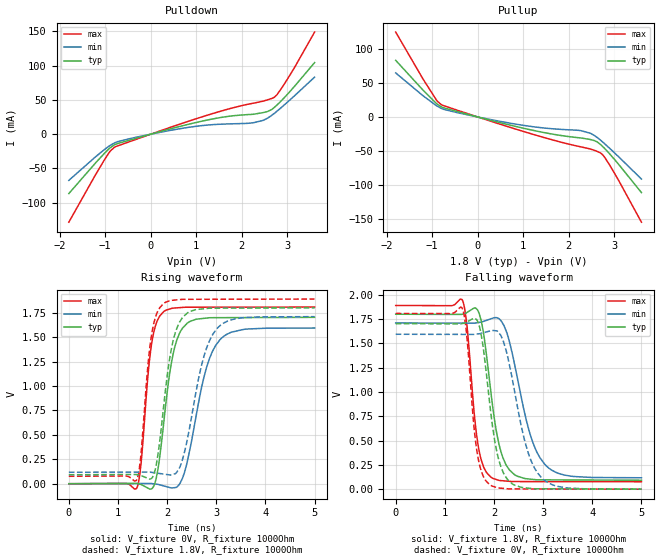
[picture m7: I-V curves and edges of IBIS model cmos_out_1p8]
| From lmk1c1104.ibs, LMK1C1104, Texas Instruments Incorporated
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[Model]   cmos_out_1p8
Model_type   Output
Polarity   Non-Inverting
Vmeas = 0.9
Vref = 0
Cref = 5pF
Rref = 100000
|   typ   min   max
C_comp   2.527pF   2.231pF   2.947pF
[Voltage Range]   1.8   1.71   1.89
[Temperature Range]   25   150   -40
[Pullup Reference]   1.8   1.71   1.89
[Pulldown Reference]   0   -0   0
[Power Clamp Reference]   1.8   1.71   1.89
[GND Clamp Reference]   0   0   0
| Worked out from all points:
|   slope of the pulldown table from 0 to 0.27 V, typ, clamps not added: 55 ohm
|   slope of the pullup table from 0 to 0.27 V, typ, clamps not added: 58.1 ohm
|   falling waveform, V_fixture 1.8V, R_fixture 1000Ohm: 20-80 % time 288ps typ, 452ps min, 202ps max; typ from 1.8 V to 0.092 V
|   rising waveform, V_fixture 0V, R_fixture 1000Ohm: 20-80 % time 272ps typ, 409ps min, 193ps max; typ from 0 V to 1.7 V
|   rising waveform, V_fixture 1.8V, R_fixture 1000Ohm: 20-80 % time 270ps typ, 402ps min, 194ps max; typ from 0.092 V to 1.8 V
|   falling waveform, V_fixture 0V, R_fixture 1000Ohm: 20-80 % time 273ps typ, 419ps min, 193ps max; typ from 1.7 V to 0 V
[Pulldown]
|   Voltage   I(typ)   I(min)   I(max)
-1.8V     -86.73mA   -67.44mA   -128.5mA
-1.012V   -27.53mA   -22.15mA   -36.77mA
-887.4mV  -19.56mA   -16.21mA   -24.46mA
-790.2mV  -15.19mA   -12.58mA   -18.76mA
840.6mV   14.63mA    10.07mA    19.14mA
1.597V    24.97mA    14.72mA    34.7mA
2.266V    29.19mA    16.87mA    45.33mA
2.471V    31.52mA    20.17mA    48.27mA
2.709V    38.7mA     30.06mA    53.65mA
2.779V    42.88mA    33.83mA    58.05mA
3.028V    59.99mA    48.17mA    83.04mA
3.6V      104.5mA    83.27mA    149mA
[Pullup]
|   Voltage   I(typ)   I(min)   I(max)
-1.8V     83.19mA    64.65mA    124.6mA
-1.184V   38.35mA    30.4mA     54.1mA
-909mV    19.99mA    16.75mA    25.25mA
-790.2mV  14.55mA    12.39mA    17.74mA
921.6mV   -15.26mA   -11.45mA   -19.57mA
1.672V    -25.54mA   -17.51mA   -34.19mA
2.266V    -30.82mA   -20.06mA   -43.89mA
2.477V    -33.13mA   -23.92mA   -47.02mA
2.709V    -40.95mA   -34.59mA   -53.22mA
2.779V    -45.48mA   -38.65mA   -58.05mA
3.006V    -62.3mA    -52.61mA   -82.49mA
3.6V      -111.1mA   -91.21mA   -154.6mA
[Ramp]
R_load = 1000
|   typ   min   max
dV/dt_r   1.02176/2.70999e-10   0.956275/4.06948e-10   1.08487/1.9283e-10
dV/dt_f   1.0249/2.88029e-10   0.955629/4.5067e-10   1.08825/2.01807e-10
[Falling Waveform]
V_fixture = 1.8V
V_fixture_min = 1.71V
V_fixture_max = 1.89V
R_fixture = 1000Ohm
C_fixture = 0F
|   Time   V(typ)   V(min)   V(max)
0s        1.8V       1.71V      1.89V
1.351ns   1.799V     1.708V     1.951V
1.447ns   1.817V     1.708V     1.695V
1.678ns   1.832V     1.714V     448.5mV
1.931ns   1.023V     1.752V     126mV
2.083ns   504.1mV    1.759V     93.59mV
2.25ns    246mV      1.624V     83.42mV
2.732ns   103.5mV    570.8mV    78.07mV
3.036ns   95.95mV    254.3mV    77.82mV
5ns       91.81mV    117.3mV    76.23mV
[Rising Waveform]
V_fixture = 0V
V_fixture_min = 0V
V_fixture_max = 0V
R_fixture = 1000Ohm
C_fixture = 0F
|   Time   V(typ)   V(min)   V(max)
0s        8.034uV    18.86uV    8.816uV
1.376ns   2.887mV    2.128mV    -50.8mV
1.467ns   -7.164mV   2.269mV    194mV
1.678ns   -53.75mV   2.067mV    1.409V
1.931ns   625.4mV    -22.55mV   1.762V
2.083ns   1.227V     -43.19mV   1.793V
2.27ns    1.558V     12.4mV     1.803V
2.78ns    1.694V     1.151V     1.807V
3.093ns   1.7V       1.483V     1.807V
5ns       1.703V     1.594V     1.808V
[Rising Waveform]
V_fixture = 1.8V
V_fixture_min = 1.71V
V_fixture_max = 1.89V
R_fixture = 1000Ohm
C_fixture = 0F
|   Time   V(typ)   V(min)   V(max)
0s        91.81mV    117.3mV    76.23mV
1.376ns   93.84mV    118.7mV    33.61mV
1.457ns   86.57mV    118.8mV    248.9mV
1.678ns   53mV       117.1mV    1.506V
1.931ns   800.3mV    98.77mV    1.845V
2.083ns   1.372V     90.15mV    1.876V
2.25ns    1.652V     160.6mV    1.885V
2.757ns   1.791V     1.319V     1.888V
3.036ns   1.797V     1.599V     1.888V
5ns       1.8V       1.71V      1.89V
[Falling Waveform]
|Gnd
V_fixture = 0V
V_fixture_min = 0V
V_fixture_max = 0V
R_fixture = 1000Ohm
C_fixture = 0F
|   Time   V(typ)   V(min)   V(max)
0s        1.703V     1.594V     1.808V
1.351ns   1.703V     1.592V     1.862V
1.436ns   1.717V     1.592V     1.629V
1.658ns   1.735V     1.596V     372.9mV
1.909ns   896.5mV    1.626V     47.31mV
2.058ns   382.4mV    1.628V     16.27mV
2.212ns   147.8mV    1.486V     6.916mV
2.626ns   14.3mV     495.4mV    2.165mV
2.959ns   3.938mV    121.7mV    1.862mV
5ns       8.033uV    18.84uV    8.817uV
